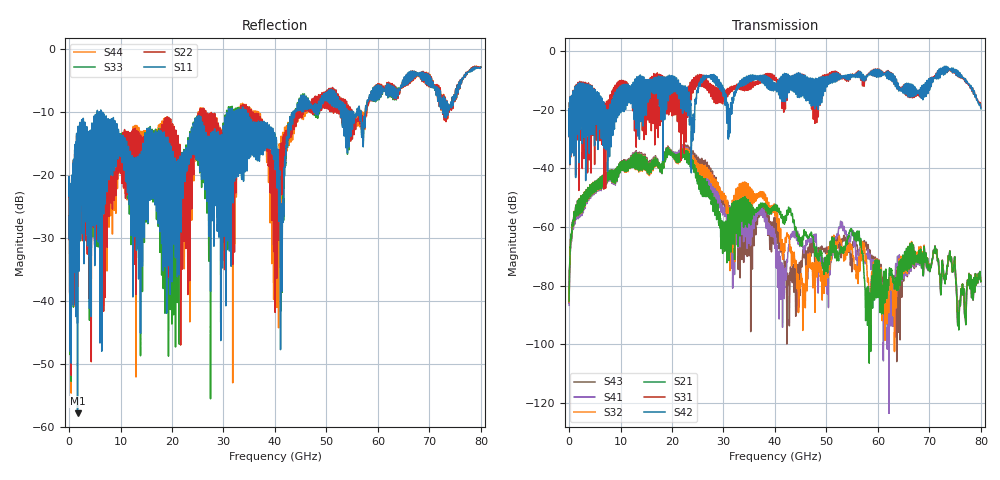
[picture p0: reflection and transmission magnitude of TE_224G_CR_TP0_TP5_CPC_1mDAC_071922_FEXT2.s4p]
!! Reference: tracy_3df_01a_2207
!! CHANNEL DESCRIPTION: TP0_TP5 CR Channel using 1meter DAC, CABLED CPC Host
!! MODEL DESCRIPTION: s4p, FEXT2
!! CONNECTOR DESCRIPTION: OSFP 200G OTB, CPC Socket
!! CABLE DESCRIPTION: 1meter 26AWG Cable
!! MODEL STATUS: Developmental
!! PORT DEFINITIONS:
!! Port  1  ----->  Side A  Side B  <-----  Port  2
!! Port  3  ----->  Side A  Side B  <-----  Port  4
# GHz S MA R 50
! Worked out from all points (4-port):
!   8000 points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, 10 MHz to 80 GHz, reference 50 ohm
!   strongest paths, dB at 10 MHz, 20.01 GHz, 40.01 GHz, 60.01 GHz, 80 GHz:
!     S42: -24.7, -13.4, -13.3, -8.7, -19.7
!     S31: -24.6, -20.2, -10.1, -8.2, -19.3
!     S21: -85.3, -35.0, -54.2, -83.5, -78.5
!     S32: -85.5, -35.0, -55.8, -77.3, -78.5
!     S41: -86.7, -34.6, -65.2, -80.0, -78.6
!     S43: -86.0, -34.3, -65.2, -74.7, -78.6
!   lowest |S11| = -57.8 dB at 1.64 GHz (marker M1), VSWR 1.00, Z = 49.9 - j0.00388 ohm
!   |S11| at or under -10 dB: start of sweep to 5.488 GHz; 6.171 GHz to 30.97 GHz (24.8 GHz wide, 134 % of centre); 34.4 GHz to 43.55 GHz (9.158 GHz wide, 23.5 % of centre)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
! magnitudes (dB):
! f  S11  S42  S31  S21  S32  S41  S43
! 10 MHz  -23.3  -24.7  -24.6  -85.3  -85.5  -86.7  -86.0
! 1.64 GHz  -57.8  -21.1  -19.6  -52.4  -52.3  -53.2  -52.6
! 22.37 GHz  -17.4  -20.1  -32.9  -33.2  -32.9  -32.2  -31.7
! 29.93 GHz  -13.4  -13.9  -14.5  -66.3  -50.3  -55.8  -52.4
! 42.57 GHz  -12.7  -9.3  -10.5  -54.6  -62.9  -68.1  -78.7
! 57.88 GHz  -8.6  -8.7  -8.3  -82.7  -75.1  -70.8  -68.0
! 80 GHz  -2.9  -19.7  -19.3  -78.5  -78.5  -78.6  -78.6
